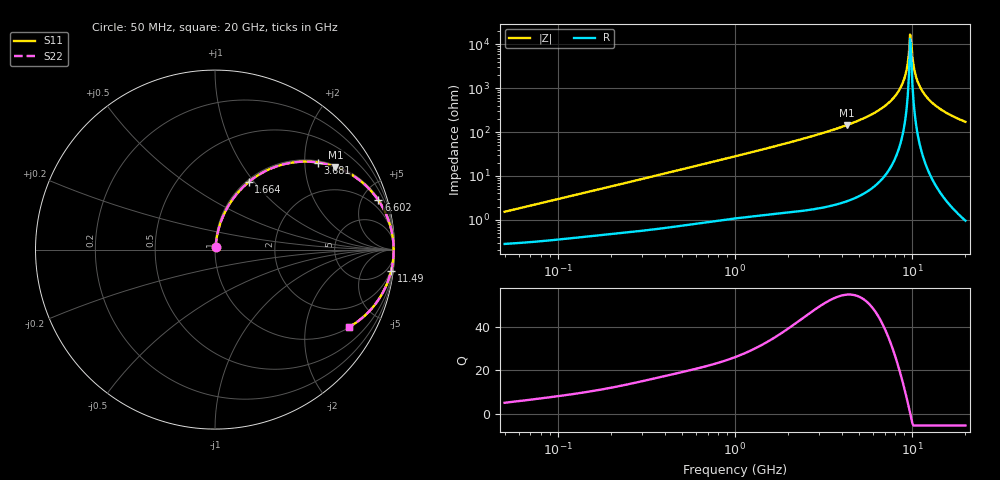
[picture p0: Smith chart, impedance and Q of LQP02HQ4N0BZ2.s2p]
!Murata Part Number: LQP02HQ4N0BZ2
!These Parameters are Measured in Series Mode Connection
!  o--[Z]--o
!Port1  Port2
!  o-------o
!Freq. Start=50[MHz] Stop=20[GHz], 401[Steps]
# Hz S RI R 50
!Freq.(Hz) S11(Real) S11(Imag) S21(Real) S21(Imag) S12(Real) S12(Imag) S22(Real) S22(Imag)
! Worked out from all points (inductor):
!   401 points, 50 MHz to 20 GHz, reference 50 ohm
!   read as one part in series: L = 4.74 nH near 51.52 MHz
!   highest Q = 54.5 at 4.276 GHz (marker M1), where L = 5.35 nH
!   self-resonance near 9.745 GHz
!   S11 on the Smith chart (normalised r, x): 50 MHz: 1.01, +0.03; 1.664 GHz: 1.03, +0.94; 3.681 GHz: 1.04, +2.33; 6.602 GHz: 1.15, +6.58; 11.49 GHz: 2, -17; 20 GHz: 1.02, -3.43
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5e7  0.00303 0.0149  0.997 -0.0149  0.997 -0.0149  0.00303 0.0149
1.364002e8  0.00557 0.0394  0.9944 -0.0394  0.9944 -0.0394  0.00557 0.0394
3.721004e8  0.017 0.1029  0.983 -0.1029  0.983 -0.1029  0.017 0.1029
1e9  0.0807 0.2539  0.9193 -0.2539  0.9193 -0.2539  0.0807 0.2539
1.664083e9  0.1875 0.3762  0.8125 -0.3762  0.8125 -0.3762  0.1875 0.3762
2.728004e9  0.3961 0.4785  0.6039 -0.4785  0.6039 -0.4785  0.3961 0.4785
3.680849e9  0.5751 0.485  0.4249 -0.485  0.4249 -0.485  0.5751 0.485
4.275624e9  0.6709 0.4608  0.3291 -0.4608  0.3291 -0.4608  0.6709 0.4608
6.601595e9  0.9101 0.2747  0.0899 -0.2747  0.0899 -0.2747  0.9101 0.2747
7.442007e9  0.9529 0.1977  0.0471 -0.1977  0.0471 -0.1977  0.9529 0.1977
8.141811e9  0.9757 0.1353  0.0243 -0.1353  0.0243 -0.1353  0.9757 0.1353
8.774992e9  0.9882 0.0812  0.0118 -0.0812  0.0118 -0.0812  0.9882 0.0812
9.178299e9  0.9927 0.0481  0.0073 -0.0481  0.0073 -0.0481  0.9927 0.0481
9.600142e9  0.995 0.0147  0.00501 -0.0147  0.00501 -0.0147  0.995 0.0147
9.745021e9  0.9953 0.00356  0.00474 -0.00356  0.00474 -0.00356  0.9953 0.00356
1.004137e10  0.995 -0.0187  0.00497 0.0187  0.00497 0.0187  0.995 -0.0187
1.034674e10  0.9938 -0.041  0.0062 0.041  0.0062 0.041  0.9938 -0.041
1.066139e10  0.9916 -0.0632  0.00844 0.0632  0.00844 0.0632  0.9916 -0.0632
1.149051e10  0.9816 -0.118  0.0184 0.118  0.0184 0.118  0.9816 -0.118
1.257102e10  0.9617 -0.1818  0.0383 0.1818  0.0383 0.1818  0.9617 -0.1818
1.417136e10  0.9223 -0.2612  0.0777 0.2612  0.0777 0.2612  0.9223 -0.2612
2e10  0.7447 -0.4333  0.2553 0.4333  0.2553 0.4333  0.7447 -0.4333
